(* Logix 5000 AddOnInstructionDefinition export AMCI_3601_AOP_Reset_Errors; software revision 20.03 *)

ADD_ON_INSTRUCTION AMCI_3601_AOP_Reset_Errors   (* revision 0.0, vendor AMCI, ExecuteEnableInFalse *)
// Revision note:
// 3/2020: Version 0 is the initial release
VAR_INPUT
   Axis_Status_Bits : INT; {required}
END_VAR
VAR_OUTPUT
   EN : BOOL; {access Read Only, visible}
   ER : BOOL; {access Read Only, visible}
END_VAR
VAR_IN_OUT
   AMCI_3601_output_data : AM:1769_3601:O:0; {required}
END_VAR
VAR
   Upper_Result_X_1000 : DINT;
   command_data_block : INT[10];
        [0]   // Command Bits MSW
        [1]   // Command Bits LSW
        [2]   // Upper Target Position
        [3]   // Lower Target Position
        [4]   // Upper Programmed Speed
        [5]   // Lower Programmed Speed
END_VAR

ROUTINE EnableInFalse   (* ladder *)
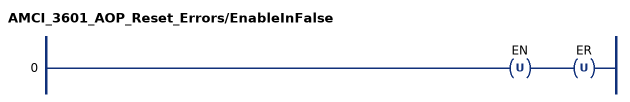
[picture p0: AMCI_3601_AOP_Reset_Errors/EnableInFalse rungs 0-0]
   0: OTU(EN)OTU(ER);
END_ROUTINE

ROUTINE Logic   (* ladder *)
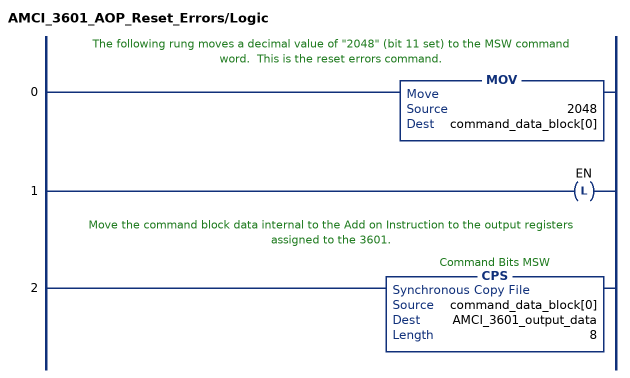
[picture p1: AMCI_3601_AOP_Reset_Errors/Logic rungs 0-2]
   // The following rung moves a decimal value of "2048" (bit 11 set) to the MSW command word.  This is the reset errors command.
   0: MOV(2048,command_data_block[0]);
   1: OTL(EN);
   // Move the command block data internal to the Add on Instruction to the output registers assigned to the 3601.
   2: CPS(command_data_block[0],AMCI_3601_output_data,8);
END_ROUTINE
END_ADD_ON_INSTRUCTION
